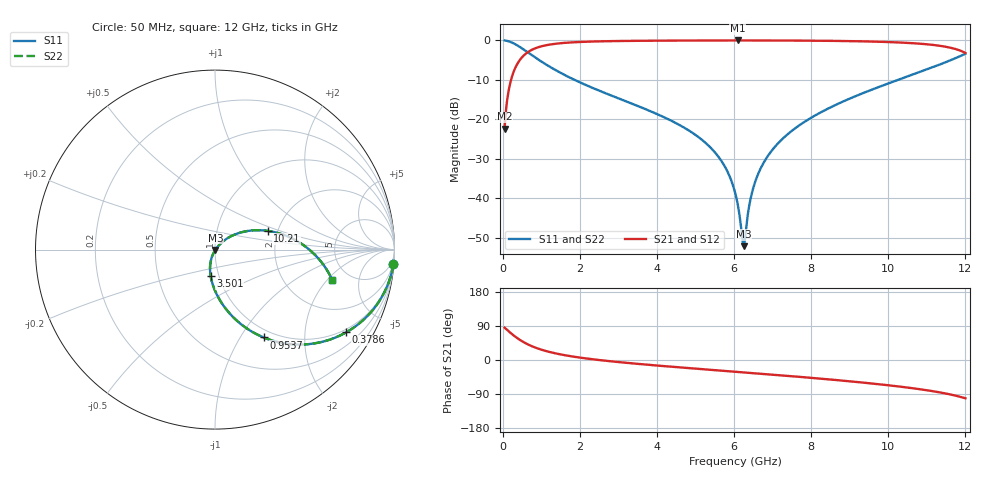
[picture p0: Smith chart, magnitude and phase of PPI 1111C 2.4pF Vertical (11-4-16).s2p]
# GHz S MA R 50
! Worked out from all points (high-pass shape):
!   1601 points, 50 MHz to 12 GHz, reference 50 ohm
!   highest |S21| = -0.02 dB at 6.1 GHz (marker M1); lowest = -22.3 dB at 50 MHz (marker M2)
!   |S21| within 3 dB of the highest: 647.2 MHz to 11.97 GHz (11.32 GHz wide, 179 % of centre)
!   lowest |S11| = -52.1 dB at 6.249 GHz (marker M3), VSWR 1.00, Z = 50.2 - j0.136 ohm
!   |S11| at or under -10 dB: 1.865 GHz to 10.26 GHz (8.391 GHz wide, 138 % of centre)
!   |S22| runs from -52.1 to 0.0 dB; largest |S21 - S12| = 0
!   S11 on the Smith chart (normalised r, x): 50 MHz: 1, -25; 378.6 MHz: 0.89, -3.24; 953.7 MHz: 0.89, -1.27; 3.501 GHz: 0.91, -0.27; 10.21 GHz: 1.77, +0.41; 12 GHz: 3.64, -2.31
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0.05  0.9971 -4.7  0.07648 85.3  0.07648 85.3  0.9971 -4.7
0.1919063  0.9592 -17.4  0.2825 72.5  0.2825 72.5  0.9592 -17.4
0.378625  0.8641 -32.2  0.5028 57.7  0.5028 57.7  0.8641 -32.2
0.6101562  0.7282 -46.5  0.6846 43.4  0.6846 43.4  0.7282 -46.5
0.9537187  0.5596 -61.0  0.8278 28.9  0.8278 28.9  0.5596 -61.0
2.044156  0.2881 -84.0  0.9562 5.8  0.9562 5.8  0.2881 -84.0
3.500563  0.1479 -99.5  0.9871 -10.2  0.9871 -10.2  0.1479 -99.5
4.038312  0.1147 -104.0  0.9913 -14.9  0.9913 -14.9  0.1147 -104.0
5.390156  0.04396 -113.0  0.9965 -25.9  0.9965 -25.9  0.04396 -113.0
5.778531  0.02443 -113.5  0.997 -28.9  0.997 -28.9  0.02443 -113.5
6.025  0.01194 -109.3  0.9972 -30.9  0.9972 -30.9  0.01194 -109.3
6.099687  0.0082 -104.2  0.9972 -31.5  0.9972 -31.5  0.0082 -104.2
6.20425  0.003424 -76.2  0.9972 -32.3  0.9972 -32.3  0.003424 -76.2
6.249062  0.002485 -33.1  0.9972 -32.7  0.9972 -32.7  0.002485 -33.1
6.480594  0.0126 43.7  0.997 -34.5  0.997 -34.5  0.0126 43.7
6.764406  0.02807 47.7  0.9965 -36.8  0.9965 -36.8  0.02807 47.7
7.264812  0.05716 46.2  0.995 -40.9  0.995 -40.9  0.05716 46.2
8.019156  0.1062 41.0  0.9906 -47.2  0.9906 -47.2  0.1062 41.0
10.01331  0.2863 22.0  0.9517 -66.8  0.9517 -66.8  0.2863 22.0
10.21497  0.311 19.6  0.9434 -69.2  0.9434 -69.2  0.311 19.6
11.29794  0.4863 3.5  0.8589 -84.8  0.8589 -84.8  0.4863 3.5
12  0.6765 -14.7  0.6936 -101.0  0.6936 -101.0  0.6765 -14.7
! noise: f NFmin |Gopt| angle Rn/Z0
0.05  0.0006377  0.9375  2.291  0.002275
1.372  0.004008  0.6936  9.208  0.002535
2.701  0.006334  0.6337  15.8  0.003194
4.031  0.008445  0.6036  22.31  0.003795
5.36  0.01054  0.5901  28.6  0.00444
6.682  0.01278  0.5898  34.58  0.005234
8.012  0.01548  0.6034  40.31  0.006401
9.341  0.01941  0.6372  45.88  0.008625
10.67  0.02796  0.7113  51.64  0.01557
12  0.07482  0.8725  58.03  0.09687
